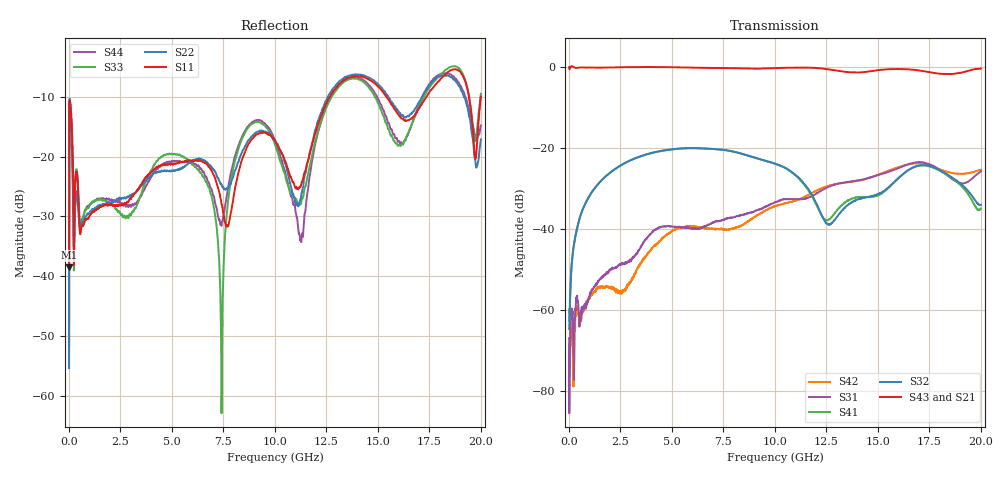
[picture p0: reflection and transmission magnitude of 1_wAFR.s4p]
!Keysight Technologies,N5225A,MY51451420,A.10.40.12
!Date: Tuesday, October 13, 2015 10:29:02
!Correction: S11(Full 4 Port(1,2,3,4))
!S12(Full 4 Port(1,2,3,4))
!S13(Full 4 Port(1,2,3,4))
!S14(Full 4 Port(1,2,3,4))
!S21(Full 4 Port(1,2,3,4))
!S22(Full 4 Port(1,2,3,4))
!S23(Full 4 Port(1,2,3,4))
!S24(Full 4 Port(1,2,3,4))
!S31(Full 4 Port(1,2,3,4))
!S32(Full 4 Port(1,2,3,4))
!S33(Full 4 Port(1,2,3,4))
!S34(Full 4 Port(1,2,3,4))
!S41(Full 4 Port(1,2,3,4))
!S42(Full 4 Port(1,2,3,4))
!S43(Full 4 Port(1,2,3,4))
!S44(Full 4 Port(1,2,3,4))
!S4P File: Measurements: <S11,S12,S13,S14>,
!<S21,S22,S23,S24>,
!<S31,S32,S33,S34>,
!<S41,S42,S43,S44>:
# Hz S  dB  R 50
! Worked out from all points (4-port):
!   2000 points, 10 MHz to 20 GHz, reference 50 ohm
!   strongest paths, dB at 10 MHz, 5.01 GHz, 10.01 GHz, 15.01 GHz, 20 GHz:
!     S43: -0.1, -0.1, -0.3, -0.8, -0.4
!     S21: -0.1, -0.1, -0.4, -1.2, -0.5
!     S32: -64.6, -20.3, -23.9, -31.4, -34.0
!     S41: -62.6, -20.4, -23.9, -31.7, -35.0
!     S31: -66.9, -39.4, -33.4, -26.7, -25.8
!     S42: -77.8, -40.5, -34.3, -26.6, -25.4
!   lowest |S11| = -38.5 dB at 10 MHz (marker M1), VSWR 1.02, Z = 51.1 - j0.363 ohm
!   |S11| at or under -10 dB: start of sweep to 12.67 GHz; 15.41 GHz to 17.36 GHz (1.956 GHz wide, 11.9 % of centre); 19.42 GHz to 20 GHz (580.7 MHz wide, 2.95 % of centre)
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1e7  -38.53 -17.4  -0.05 0.3  -67.30 -158.8  -65.45 131.9
     -0.07 0.4  -55.38 110.4  -67.38 140.4  -66.25 -161.9
     -66.88 94.4  -64.61 30.4  -36.94 -10.9  -0.10 0.5
     -62.63 72.8  -77.83 171.7  -0.10 0.1  -51.54 -12.1
7.8e8  -30.65 43.6  -0.18 -1.5  -58.88 108.6  -33.90 87.8
       -0.19 -1.5  -30.16 63.4  -33.92 88.3  -59.12 120.8
       -59.03 108.5  -33.93 88.3  -28.94 45.6  -0.20 -1.8
       -33.92 87.9  -58.89 121.7  -0.18 -1.7  -29.02 72.9
3.82e9  -23.11 -13.7  -0.06 -0.6  -42.05 57.2  -21.53 88.6
        -0.07 -0.5  -23.73 -175.3  -21.50 89.3  -46.07 -106.8
        -41.99 57.3  -21.51 89.2  -23.50 -27.3  -0.07 -2.0
        -21.53 88.7  -46.11 -105.8  -0.05 -2.0  -24.38 -166.9
7.41e9  -27.99 -104.8  -0.33 -2.4  -37.84 -79.8  -20.43 86.2
        -0.33 -2.2  -24.76 -55.4  -20.42 87.1  -39.96 -119.0
        -37.86 -79.7  -20.43 87.0  -62.94 -127.1  -0.32 -5.3
        -20.44 86.4  -39.96 -118.5  -0.30 -5.2  -31.59 -22.4
8.82e9  -17.42 73.9  -0.41 -8.7  -35.97 159.7  -22.13 80.0
        -0.42 -8.4  -16.87 81.0  -22.08 81.0  -37.71 174.6
        -35.97 160.0  -22.08 80.8  -14.72 67.9  -0.48 -12.0
        -22.13 80.2  -37.76 174.4  -0.46 -11.9  -14.51 83.9
1.127e10  -24.80 17.3  -0.23 -11.6  -32.66 -1.9  -28.15 79.5
          -0.23 -11.3  -26.73 123.9  -27.92 79.4  -32.46 168.0
          -32.67 -1.5  -27.93 79.4  -27.85 -35.6  -0.20 -15.6
          -28.13 79.9  -32.44 168.2  -0.19 -15.5  -34.13 175.7
2e10  -9.98 -75.9  -0.52 -28.7  -25.79 131.4  -34.91 -88.8
      -0.53 -28.1  -17.11 -91.1  -34.02 -98.5  -25.39 -2.0
      -25.77 131.5  -34.04 -98.8  -9.51 -84.5  -0.44 -37.0
      -34.95 -88.4  -25.38 -2.0  -0.42 -36.7  -14.81 -84.5
